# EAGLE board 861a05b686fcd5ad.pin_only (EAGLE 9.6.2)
REV: C

Size 25.4 x 17.78 mm. Coordinates in mm from the lower left corner, seen from the top.
Outline: 0,2.54 0,15.24 arc-90 2.54,17.78 22.86,17.78 arc-90 25.4,15.24 25.4,2.54 arc-90 22.86,0 2.54,0 arc-90 0,2.54
Copper layers (1*16): Top 0.035mm / dielectric 1.5mm / Bottom 0.035mm
Design rules "adafruit": minimum track width 8mil, minimum drill 15.5mil, track to track 8mil, track to pad 8mil, pad to pad 8mil, via to via 8mil, smd to smd 8mil, copper to edge 10mil, drill to drill 8mil, minimum pad ring 10mil, minimum via ring 8mil, stop-mask expansion 2mil, vias tented up to drill 20mil, thermal gap 10mil

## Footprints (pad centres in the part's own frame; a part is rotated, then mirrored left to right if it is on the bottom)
0603-NO = smd 1.075 x 1: 1 -0.85,0; 2 0.85,0
0805-NO = smd 1.24 x 1.5: 1 -0.95,0; 2 0.95,0
FIDUCIAL_1MM = smd 1 x 1: 1 0,0
1X09_ROUND_70 = drill 1 pad 1.778: 1 -10.16,0; 2 -7.62,0; 3 -5.08,0; 4 -2.54,0; 5 0,0; 6 2.54,0; 7 5.08,0; 8 7.62,0; 9 10.16,0
RESPACK_4X0603 = smd 0.45 x 0.9: 1 -1.3,-0.85; 2 -0.4,-0.85; 3 0.4,-0.85; 4 1.3,-0.85; 5 1.3,0.85; 6 0.4,0.85; 7 -0.4,0.85; 8 -1.3,0.85
SOIC8_208MIL = smd 0.6 x 2.2: 1 -1.905,-3.315; 2 -0.635,-3.315; 3 0.635,-3.315; 4 1.905,-3.315; 5 1.905,3.315; 6 0.635,3.315; 7 -0.635,3.315; 8 -1.905,3.315
USON8 = smd 0.5 x 0.275: 1 -1.2,0.75; 2 -1.2,0.25; 3 -1.2,-0.25; 4 -1.2,-0.75; 5 1.2,-0.75; 6 1.2,-0.25; 7 1.2,0.25; 8 1.2,0.75
TSSOP16 = smd 0.305 x 0.991: 1 -2.275,-2.918; 2 -1.625,-2.918; 3 -0.975,-2.918; 4 -0.325,-2.918; 5 0.325,-2.918; 6 0.975,-2.918; 7 1.625,-2.918; 8 2.275,-2.918; 9 2.275,2.918; 10 1.625,2.918; 11 0.975,2.918; 12 0.325,2.918; 13 -0.325,2.918; 14 -0.975,2.918; 15 -1.625,2.918; 16 -2.275,2.918
SOT23-5 = smd 0.55 x 1.2: 1 -0.95,-1.3; 2 0,-1.3; 3 0.95,-1.3; 4 0.95,1.3; 5 -0.95,1.3
MOUNTINGHOLE_2.5_PLATED = drill 2.5 pad 3.2: P$1 0,0

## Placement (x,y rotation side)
C1  0.1uF  [0603-NO]  15.24,5.46 0 top
C3  10uF  [0805-NO]  3.43,11.68 0 top
C4  10uF  [0805-NO]  3.56,6.35 0 top
FID2  FIDUCIAL_1MM  [FIDUCIAL_1MM]  0.89,6.73 0 top
FID3  FIDUCIAL_1MM  [FIDUCIAL_1MM]  24.13,10.41 0 top
JP1  [1X09_ROUND_70]  12.7,2.54 180 top
R1  10K  [RESPACK_4X0603]  23.11,7.24 90 top
U1  Generic SPI Flash  [SOIC8_208MIL]  15.24,8.64 90 top
U2  Generic SPI Flash  [USON8]  15.24,12.7 180 top
U3  74HC4050D  [TSSOP16]  8,9.02 0 top
U4  AP2112K-3.3  [SOT23-5]  3.17,9.02 270 top
U$16  MOUNTINGHOLE2.5  [MOUNTINGHOLE_2.5_PLATED]  2.54,15.24 0 top
U$17  MOUNTINGHOLE2.5  [MOUNTINGHOLE_2.5_PLATED]  22.86,15.24 0 top
U$19  [ADAFRUIT_3.5MM]  4.83,13.59 0 top
U$21  [PCBFEAT-REV-040]  5.84,16.26 0 bottom

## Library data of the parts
C1 C3 C4 JP1 R1 U1-U4 U$19 = microbuilder
FID2 FID3 U$16 U$17 = microbuilder; BOM: EXCLUDE
U$21 = microbuilder; REV: C

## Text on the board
tPlace: SPI FRAM | VIN | GND | MISO | CS | !Hold | 3V3 | SCK | MOSI | !WP
bPlace: SPI FRAM | Model/Capacity: | Vin/Vlogic: 3~5V

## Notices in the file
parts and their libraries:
microbuilder: This work is placed in the public domain, and may be freely used for commercial and non-commercial work with the following conditions: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
